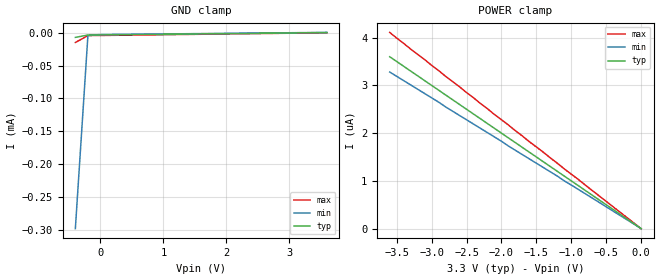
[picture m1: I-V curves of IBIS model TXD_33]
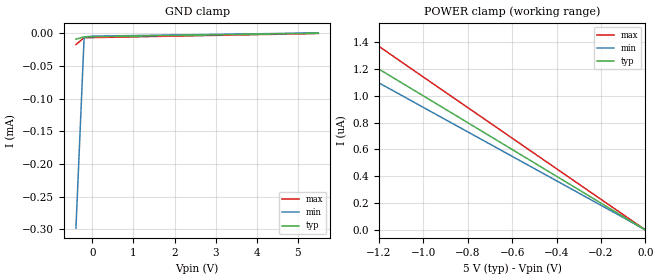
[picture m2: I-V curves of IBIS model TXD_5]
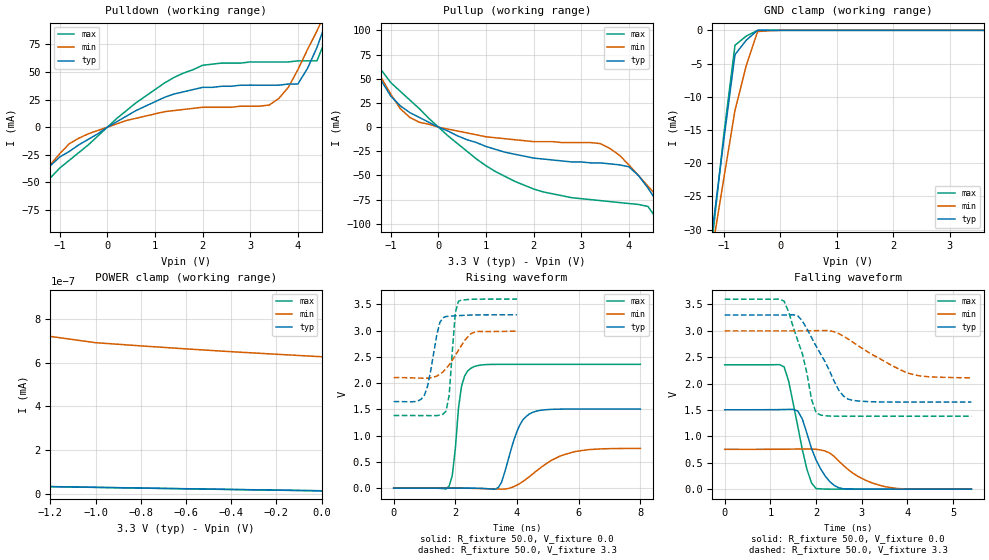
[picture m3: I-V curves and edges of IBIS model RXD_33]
|Texas Instruments Incorporated
[IBIS Ver]   4.1
[File name]   iso6163dw.ibs
[File Rev]   1.0
[Date]   02/17/2025
[Source]   Model built from TISPICED simulations at:
   Texas Instruments Incorporated.
   Analog-eLab, HPA
   12500 TI Blvd
   Dallas, TX -75243
   For Support e-mail: elab_ibis@list.ti.com
[Notes]   Revision History
   Rev 1.0: 02/17/2025
   - Model based on ISO7241
   - C_comp although listed in numberical order of value are obtained from varying PVT conditions.
   For PVT conditions for eachspecific value, refer to the buffer description under repective [Model].
   IBIS model user is responsible for using appropriate C_comp to simulate for Signal Integrity.
[Disclaimer] This product is designed as an aid for customers of Texas
   Instruments.
   No warranties, either expressed or implied, with respect
   to this third party software (if any) or with respect to
   its fitness for any particular purpose is claimed by Texas
   Instruments or the author. The software (if any) is provided
   solely on an "as is" basis. The entire risk as to its quality
   and performance is with the customer
[Copyright]   (C)Copyright 2025 Texas Instruments Incorporated.
   All rights reserved.
|   ISO6163DW
[Component]   ISO6163DW
[Manufacturer]   Texas Instruments Incorporated
[Package]   |16 SOIC - DW package
|   typ   min   max
R_pkg   0.13983   0.12494   0.17928
L_pkg   2.1802nH   1.92454nH   2.85707nH
C_pkg   0.42060pF   0.21450pF   0.61276pF
[Pin]  signal_name   model_name   R_pin   L_pin   C_pin
1   VCC1   POWER   0.09703   2.25823nH  0.63889pF
2   INA   TXD1   0.10567   2.15194nH  0.30706pF
3   INB   TXD1   0.12889   1.99554nH  0.21450pF
4   INC   TXD1   0.12623   1.94755nH  0.61276pF
5   OUTD   RXD1   0.12494   1.92646nH  0.36666pF
6   OUTE   RXD1   0.14038   2.18765nH  0.43235pF
7   OUTF   RXD1   0.06469   1.55584nH  0.24569pF
8   GND1   GND   0.08216   2.43955nH  0.44498pF
9   GND2   GND   0.10126   2.44074nH  0.40934pF
10   INF   TXD2   0.17928   2.85707nH  0.52717pF
11   INE   TXD2   0.12883   1.99615nH  0.50841pF
12   IND   TXD2   0.12617   1.94399nH  0.32633pF
13   OUTC   RXD2   0.12498   1.92454nH  0.37783pF
14   OUTB   RXD2   0.14050   2.18615nH  0.38097pF
15   OUTA   RXD2   0.08275   2.09014nH  0.75096pF
16   VCC2   POWER   0.09747   2.26909nH  0.67439pF
|   Model Selectors
[Model Selector] TXD1
TXD_33   TXD Input model for 3.0V - 3.6V
TXD_5   TXD Input model for 4.5V - 5.5V
[Model Selector] RXD1
RXD_33   RXD Output model for 3.0V - 3.6V
RXD_5   RXD Output model for 4.5V - 5.5V
[Model Selector] TXD2
TXD_33   TXD Input model for 3.0V - 3.6V
TXD_5   TXD Input model for 4.5V - 5.5V
[Model Selector] RXD2
RXD_33   RXD Output model for 3.0V - 3.6V
RXD_5   RXD Output model for 4.5V - 5.5V|
| Models and submodels in the file (4): TXD_33 (Input), TXD_5 (Input), RXD_33 (3-state), RXD_5 (3-state)
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|   TXD_33 Model
[Model]   TXD_33
Model_type   Input
|Signals   TXD
Vinh = 2.0
Vinl = 0.8
|   typ   min   max
C_comp   1.3pF   1.1pF   1.5pF
|   typ   min   max
[Temperature Range]   27   -40   125
[Voltage range]   3.3V   3.0V   3.6V
[GND_clamp]
|   Voltage   I(typ)   I(min)   I(max)
-400mV    -7.04uA    -298uA     -14.8uA
-200mV    -3.5uA     -3.91uA    -4.34uA
0V        -3.3uA     -2.74uA    -4.11uA
3.6V      300nA      549nA      14.4pA
[Power_clamp]
| Note that the[POWER_clamp]voltage table is referenced to Vcc
| and is calculated using Vtable=Vcc - Vmeasured.
|   Voltage   I(typ)   I(min)   I(max)
-3.6V     3.6uA      3.28uA     4.11uA
-2.9V     2.9uA      2.65uA     3.31uA
-2.8V     2.8uA      2.55uA     3.19uA
0V        0A         0A         0A
|   TXD_5 Model
[Model]   TXD_5
Model_type   Input
|Signals   TXD
Vinh = 2.0
Vinl = 0.8
|   typ   min   max
C_comp   1.3pF   1.1pF   1.5pF
|   typ   min   max
[Temperature Range]   27   -40   125
[Voltage range]   5.0V   4.5V   5.5V
[GND_clamp]
|   Voltage   I(typ)   I(min)   I(max)
-400mV    -8.71uA    -298uA     -16.9uA
-200mV    -5.2uA     -5.27uA    -6.5uA
0V        -5uA       -4.1uA     -6.27uA
5.5V      500nA      913nA      27.5pA
[Power_clamp]
| Note that the[POWER_clamp]voltage table is referenced to Vcc
| and is calculated using Vtable=Vcc - Vmeasured.
|   Voltage   I(typ)   I(min)   I(max)
-5.5V     5.498uA    5.021uA    6.28uA
-1.7V     1.699uA    1.552uA    1.939uA
-1.6V     1.599uA    1.461uA    1.825uA
-1.5V     1.499uA    1.369uA    1.711uA
-1.4V     1.399uA    1.278uA    1.597uA
-1.3V     1.299uA    1.187uA    1.483uA
0V        0A         0A         0A
[Model]   RXD_33
Model_type   3-state
| Signals   RXD
Vmeas = 2.2V   |Reference voltage for timing measurements
Cref = 15pF   |Timing specification test load capacitance value
Vref = 0   |Timing specification test load voltage; GND
| variable   typ   min   max
C_comp   2.1pF   1.7pF   2.5pF
|   typ   min   max
[Temperature Range]   25.0   -40   125
[Voltage range]   3.3V   3.0V   3.6V
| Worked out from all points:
|   slope of the pulldown table from 0 to 0.495 V, typ, clamps not added: 40 ohm
|   slope of the pullup table from 0 to 0.495 V, typ, clamps not added: 45.4 ohm
|   GND clamp passes 1 mA (typ) near -0.54 V on its own axis
|   POWER clamp passes 1 mA (typ) near -2.27 V on its own axis
|   rising waveform, R_fixture 50.0, V_fixture 0.0: 20-80 % time 494ps typ, 1.13ns min, 242ps max; typ from 0 V to 1.5 V
|   falling waveform, R_fixture 50.0, V_fixture 0.0: 20-80 % time 416ps typ, 716ps min, 336ps max; typ from 1.5 V to 0 V
|   rising waveform, R_fixture 50.0, V_fixture 3.3: 20-80 % time 308ps typ, 597ps min, 168ps max; typ from 1.65 V to 3.3 V
|   falling waveform, R_fixture 50.0, V_fixture 3.3: 20-80 % time 592ps typ, 1.04ns min, 405ps max; typ from 3.3 V to 1.65 V
[Pulldown]
|   Voltage  I(typ)   I(min)   I(max)
-3.6V     -213mA     -167mA     -286mA
-2.2V     -106mA     -89mA      -137mA
-1.8V     -76mA      -66mA      -95mA
-1.2V     -35mA      -34mA      -46mA
-600mV    -16mA      -10mA      -23mA
2V        36mA       18mA       56mA
3.4V      38mA       20mA       59mA
4V        39mA       52mA       60mA
4.4V      72mA       87mA       60mA
4.6V      96mA       106mA      81mA
4.8V      120mA      124mA      106mA
7.5V      465mA      379mA      575mA
[Pullup]
|   Voltage   I(typ)  I(min)  I(max)
| Note that the[Pullup]voltage table is referenced to Vcc
| and is calculated using Vtable=Vcc - Vmeasured.
-3.6V     345mA      272mA      457mA
-2V       144mA      123mA      182mA
-1.5V     83mA       78mA       100mA
-1.2V     48mA       51mA       59mA
-600mV    15mA       10mA       28mA
800mV     -16mA      -8mA       -33mA
2V        -32mA      -15mA      -64mA
3.4V      -37mA      -17mA      -76mA
4V        -41mA      -39mA      -79mA
4.4V      -63mA      -61mA      -82mA
5V        -108mA     -95mA      -134mA
7.2V      -281mA     -221mA     -373mA
[GND_clamp]
|   Voltage   I(typ)   I(min)   I(max)
| Outputs in High Impedance (off)
-3.6V     -213mA     -167.2mA   -285.4mA
-1.2V     -30.16mA   -32.94mA   -31.43mA
-1.1V     -23.41mA   -27.68mA   -23.65mA
-1V       -16.66mA   -22.42mA   -15.87mA
-800mV    -3.66mA    -12.05mA   -2.249mA
-600mV    -1.479mA   -5.279mA   -861.1uA
-400mV    -1.657uA   -187.7uA   -4.797uA
0V        -40.79pA   -10.95nA   -39.6pA
3.6V      17.57pA    663pA      12.68pA
[POWER_clamp]
|   Voltage  I(typ)   I(min)   I(max)
| Note that the [POWER_clamp] voltage table is referenced to Vcc
| and is calculated using Vtable = Vcc - Vmeasured.
| Outputs in Tri-state.
-3.6V     130.9mA    132.2mA    129.3mA
-2.2V     594.7uA    10.13mA    942.3pA
-2.1V     8.158nA    6.126mA    495.1pA
-2V       5.434nA    2.119mA    47.98pA
-1.8V     1.376nA    388.9uA    43.35pA
-1.7V     41.24pA    194.6uA    41.32pA
-1.5V     37.53pA    132.3nA    37.35pA
-1.4V     35.76pA    755.1pA    35.42pA
-1.2V     32.25pA    720.1pA    31.79pA
-1V       28.85pA    691.4pA    28.37pA
-400mV    19.15pA    650.1pA    18.72pA
0V        12.94pA    627pA      12.68pA
[Ramp]
|   typ   min   max
dV/dt_r   0.903V/0.494ns   0.454V/1.13ns   1.414V/0.242ns
dV/dt_f   0.980V/0.416ns   0.540V/0.717ns  1.333V/0.336ns
R_load = 50
[Rising Waveform]
R_fixture = 50.0
V_fixture = 0.0
C_fixture = 0p
L_fixture = 0n
|   V(typ)   V(min)   V(max)
0s        489.7pV    12.09nV    431.9pV
1.8ns     17.01uV    282.3uV    42.76mV
1.9ns     27.86uV    217.4uV    238.3mV
2.2ns     89.93uV    -788.4uV   1.94V
2.6ns     -99.63uV   -4.419mV   2.312V
3.4ns     15.91mV    -17.3mV    2.357V
4ns       1.083V     58.82mV    2.357V
4.5ns     1.441V     266mV      2.357V
5.9ns     1.506V     698.7mV    2.357V
8ns       1.505V     756mV      2.357V
[Falling Waveform]
R_fixture = 50.0
V_fixture = 0.0
C_fixture = 0p
L_fixture = 0n
|   V(typ)   V(min)   V(max)
0s        1.505V     755.2mV    2.357V
1.3ns     1.51V      757.4mV    2.318V
1.4ns     1.512V     758.3mV    2.047V
1.6ns     1.481V     760.6mV    1.187V
1.8ns     1.057V     762mV      375.6mV
2ns       553.1mV    755.1mV    12.03mV
2.3ns     143.1mV    683mV      796.9uV
2.6ns     7.515mV    447.7mV    36.71uV
3.5ns     197.3uV    48.97mV    -2.819uV
5.4ns     -4.04uV    324.3uV    303.2nV
[Rising Waveform]
R_fixture = 50.0
V_fixture = 3.3
V_fixture_min = 3.0
V_fixture_max = 3.6
C_fixture = 0p
L_fixture = 0n
|   V(typ)   V(min)  V(max)
0s        1.649V     2.106V     1.383V
1ns       1.774V     2.093V     1.382V
1.1ns     1.943V     2.094V     1.382V
1.5ns     3.156V     2.171V     1.389V
1.7ns     3.268V     2.277V     1.468V
1.8ns     3.274V     2.348V     1.768V
2ns       3.282V     2.527V     3.341V
2.1ns     3.285V     2.625V     3.559V
2.6ns     3.296V     2.964V     3.597V
4ns       3.3V       2.989V     3.6V
[Falling Waveform]
R_fixture = 50.0
V_fixture = 3.3
V_fixture_min = 3.0
V_fixture_max = 3.6
C_fixture = 0p
L_fixture = 0n
|   V(typ)   V(min)  V(max)
0s        3.3V       3V         3.6V
1.3ns     3.3V       3V         3.563V
1.6ns     3.286V     3V         2.812V
1.7ns     3.187V     3V         2.569V
1.9ns     2.874V     3.002V     1.705V
2.1ns     2.561V     3.006V     1.404V
2.5ns     1.872V     2.947V     1.383V
2.7ns     1.707V     2.846V     1.383V
4ns       1.65V      2.201V     1.383V
5.4ns     1.65V      2.11V      1.383V
